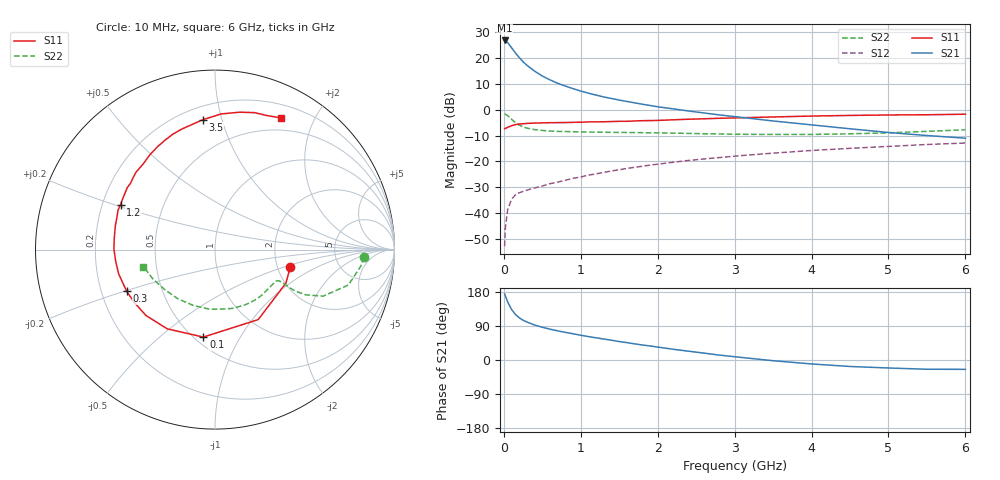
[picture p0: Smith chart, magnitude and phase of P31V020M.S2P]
! SIEMENS Small Signal Semiconductors
! BFP181
! Si NPN RF Bipolar Junction Transistor in SOT143
! VCE = 1 V  IC = 20 mA
! Common Emitter S-Parameters:  March  1996
# GHz  S  MA  R  50
!  f  S11  S21  S12  S22
! GHz  MAG  ANG  MAG  ANG  MAG  ANG  MAG  ANG
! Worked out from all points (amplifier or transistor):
!   36 points, 10 MHz to 6 GHz, reference 50 ohm
!   highest |S21| = 26.8 dB at 10 MHz (marker M1)
!   |S21| within 3 dB of that: start of sweep to 104.8 MHz
!   unconditionally stable (mu >= 1): start of sweep to 26.31 MHz; 207.2 MHz to end of sweep
!   at 250 MHz: K = 1.15, MAG = 22.7 dB, |S12| = -31.6 dB
!   at 1.4 GHz: K = 2.43, MAG = 7.3 dB, |S12| = -23.7 dB
!   at 6 GHz: K = 2.17, MAG = -5.2 dB, |S12| = -12.9 dB
!   S11 on the Smith chart (normalised r, x): 10 MHz: 2.36, -0.55; 100 MHz: 0.55, -0.71; 300 MHz: 0.31, -0.20; 1.2 GHz: 0.28, +0.21; 3.5 GHz: 0.28, +0.87; 6 GHz: 0.35, +1.56
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0.01  0.4306 -12.8  21.95 174.4  0.0023 72.7  0.8305 -2.9
0.02  0.4371 -25.3  21.74 169.0  0.0053 75.9  0.8186 -6.3
0.05  0.4583 -58.3  20.03 153.2  0.0117 66.9  0.7697 -14.8
0.1  0.4917 -97.6  15.88 133.5  0.0185 52.5  0.656 -23.3
0.15  0.5155 -121.1  12.64 120.3  0.0226 46.6  0.5645 -26.5
0.2  0.5318 -136.4  10.26 111.5  0.0248 43.1  0.5062 -27.3
0.25  0.5375 -146.8  8.505 104.9  0.0264 41.9  0.4677 -27.1
0.3  0.5442 -154.7  7.267 100.2  0.0279 41.6  0.4427 -26.6
0.4  0.5536 -165.9  5.599 92.3  0.0308 43.5  0.4138 -26.0
0.5  0.5574 -173.6  4.502 86.4  0.0336 44.4  0.3982 -26.0
0.6  0.5629 179.8  3.797 81.4  0.0372 47.1  0.3884 -26.5
0.7  0.5645 174.5  3.25 76.9  0.0399 48.9  0.3824 -27.5
0.8  0.5669 169.9  2.878 72.9  0.0434 50.4  0.379 -28.7
1.1  0.5832 157.9  2.098 61.8  0.0544 52.8  0.3713 -33.5
1.2  0.5833 154.5  1.924 58.6  0.0577 52.9  0.369 -35.4
1.7  0.6079 138.4  1.363 42.6  0.0771 53.0  0.3628 -45.7
2.2  0.6403 124.7  1.043 28.4  0.0966 50.9  0.3532 -57.6
2.8  0.6848 110.0  0.797 13.0  0.119 46.6  0.3416 -73.6
3.5  0.7263 95.5  0.608 -1.9  0.1451 40.8  0.3337 -94.7
4.5  0.7778 79.8  0.429 -17.1  0.1797 31.4  0.3432 -126.9
5.5  0.8018 68.4  0.318 -24.4  0.213 21.9  0.3829 -154.9
6  0.8212 63.4  0.282 -24.7  0.2274 16.8  0.4106 -166.7
